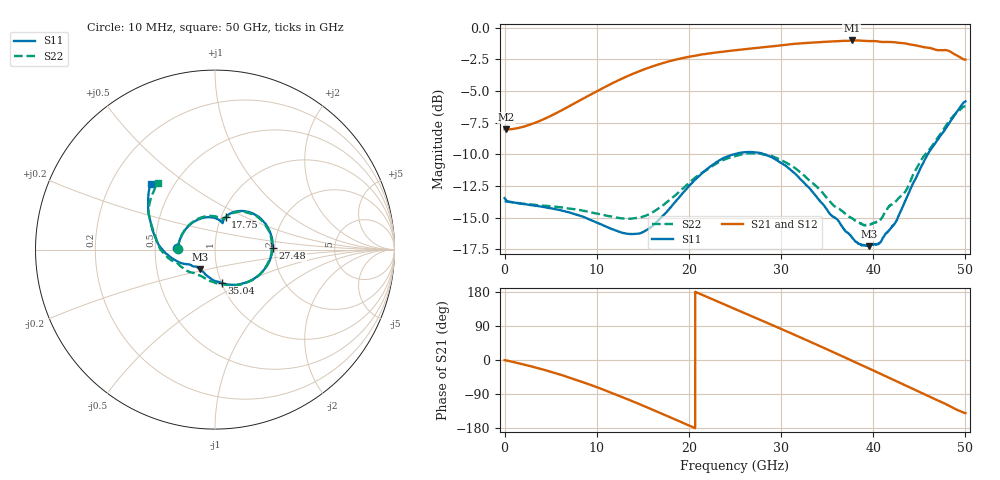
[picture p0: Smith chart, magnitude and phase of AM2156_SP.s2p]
!Keysight Technologies,N5245B,MY58422270,A.16.20.02
!Date: Wednesday, March 11, 2026 23:29:36
!Correction: S11(C  2-Port  )
!S21(C  2-Port  )
!S12(C  2-Port  )
!S22(C  2-Port  )
!S2P File: Measurements: S11, S21, S12, S22:
# Hz S  dB  R 50
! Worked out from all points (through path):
!   6401 points, 10 MHz to 50 GHz, reference 50 ohm
!   highest |S21| = -1.00 dB at 37.67 GHz (marker M1); lowest = -8.0 dB at 197.5 MHz (marker M2)
!   group delay of S21, straight-line fit = 28.7 ps
!   lowest |S11| = -17.2 dB at 39.51 GHz (marker M3), VSWR 1.32, Z = 41.4 - j9.22 ohm
!   |S11| at or under -10 dB: start of sweep to 24.8 GHz; 28.17 GHz to 45.9 GHz (17.73 GHz wide, 47.9 % of centre)
!   |S22| runs from -15.6 to -6.2 dB; largest |S21 - S12| = 0.0052
!   S11 on the Smith chart (normalised r, x): 10 MHz: 0.65, +0.01; 17.75 GHz: 1.05, +0.39; 27.48 GHz: 1.95, +0.04; 35.04 GHz: 1.00, -0.39; 50 GHz: 0.37, +0.37
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1e7  -13.45 177.6  -8.02 -0.6  -8.13 -0.2  -13.69 179.7
1.974625e8  -13.64 177.0  -8.03 -1.2  -8.06 -1.1  -13.71 177.7
5.141786e9  -14.26 122.7  -6.91 -31.9  -6.91 -31.9  -14.10 125.1
8.34427e9  -14.87 95.5  -5.66 -57.0  -5.67 -57.0  -14.42 99.1
1.296835e10  -16.21 74.8  -3.94 -99.7  -3.94 -99.7  -15.06 76.9
1.667854e10  -15.21 73.9  -2.90 -137.5  -2.90 -137.5  -14.27 70.6
1.774864e10  -14.41 72.0  -2.67 -148.8  -2.67 -148.8  -13.68 68.1
1.958421e10  -12.86 64.9  -2.35 -168.3  -2.35 -168.2  -12.53 61.4
2.135729e10  -11.52 54.2  -2.11 172.9  -2.11 173.0  -11.49 52.2
2.313038e10  -10.54 40.9  -1.94 154.2  -1.93 154.3  -10.66 40.6
2.5005e10  -9.97 24.9  -1.77 134.6  -1.77 134.6  -10.13 26.6
2.748107e10  -9.86 1.7  -1.58 108.6  -1.58 108.6  -9.93 6.1
3.045703e10  -10.87 -28.7  -1.34 77.3  -1.35 77.3  -10.61 -22.2
3.333927e10  -12.89 -59.8  -1.17 46.2  -1.16 46.2  -12.22 -51.3
3.504205e10  -14.43 -78.8  -1.09 27.6  -1.09 27.7  -13.51 -69.3
3.767434e10  -16.55 -110.3  -1.00 -1.4  -1.00 -1.3  -15.03 -98.6
3.950991e10  -17.24 -127.3  -1.05 -22.0  -1.04 -21.9  -15.51 -118.2
4.167354e10  -16.03 -146.2  -1.12 -46.1  -1.11 -46.0  -14.13 -143.4
4.364971e10  -13.37 -161.3  -1.25 -68.9  -1.26 -68.9  -12.74 -162.5
4.581334e10  -10.11 175.8  -1.56 -93.2  -1.56 -93.1  -9.86 173.7
4.843781e10  -7.31 149.5  -1.91 -123.7  -1.91 -123.7  -7.16 147.2
5e10  -5.81 134.3  -2.51 -140.1  -2.55 -140.2  -6.19 130.7
